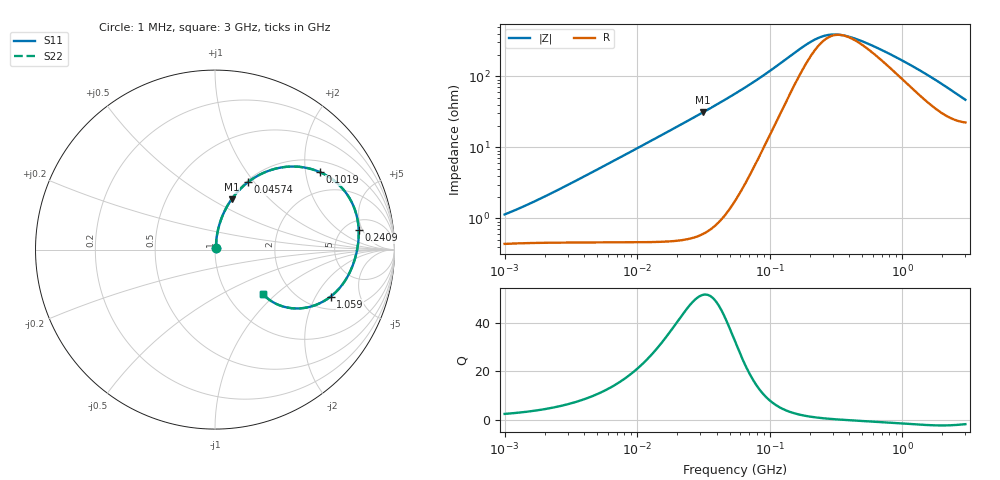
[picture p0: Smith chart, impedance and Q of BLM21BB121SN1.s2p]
! BLM21BB121SN1
# Hz S RI R 50
!Freq.(Hz) S11(Real) S11(Imag) S21(Real) S21(Imag) S12(Real) S12(Imag) S22(Real) S22(Imag)
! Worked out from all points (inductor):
!   401 points, 1 MHz to 3 GHz, reference 50 ohm
!   read as one part in series: L = 159 nH near 1.323 MHz
!   highest Q = 51.5 at 31.27 MHz (marker M1), where L = 158 nH
!   self-resonance near 349.5 MHz
!   S11 on the Smith chart (normalised r, x): 1 MHz: 1.01, +0.02; 45.74 MHz: 1.02, +0.93; 101.9 MHz: 1.32, +2.41; 240.9 MHz: 6.75, +4.21; 1.059 GHz: 2.65, -2.69; 3 GHz: 1.45, -0.82
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1000000  0.00447 0.0104  0.9955 -0.0104  0.9955 -0.0104  0.00447 0.0104
1716745  0.00479 0.0169  0.9952 -0.0169  0.9952 -0.0169  0.00479 0.0169
3823119  0.00593 0.0368  0.9941 -0.0368  0.9941 -0.0368  0.00593 0.0368
8017732  0.0105 0.0766  0.9895 -0.0766  0.9895 -0.0766  0.0105 0.0766
1.461624e7  0.0242 0.138  0.9758 -0.138  0.9758 -0.138  0.0242 0.138
3.127247e7  0.0921 0.2796  0.9079 -0.2796  0.9079 -0.2796  0.0921 0.2796
4.574308e7  0.1838 0.3757  0.8162 -0.3757  0.8162 -0.3757  0.1838 0.3757
5.477226e7  0.2512 0.4185  0.7488 -0.4185  0.7488 -0.4185  0.2512 0.4185
7.697298e7  0.4241 0.4628  0.5759 -0.4628  0.5759 -0.4628  0.4241 0.4628
1.018679e8  0.5852 0.4314  0.4148 -0.4314  0.4148 -0.4314  0.5852 0.4314
1.460522e8  0.7381 0.3042  0.2619 -0.3042  0.2619 -0.3042  0.7381 0.3042
2.094008e8  0.7958 0.1576  0.2042 -0.1576  0.2042 -0.1576  0.7958 0.1576
2.408952e8  0.8007 0.1084  0.1993 -0.1084  0.1993 -0.1084  0.8007 0.1084
3.002264e8  0.7982 0.041  0.2018 -0.041  0.2018 -0.041  0.7982 0.041
3.741707e8  0.7884 -0.0174  0.2116 0.0174  0.2116 0.0174  0.7884 -0.0174
5.051982e8  0.7667 -0.0899  0.2333 0.0899  0.2333 0.0899  0.7667 -0.0899
8.005644e8  0.7072 -0.1982  0.2928 0.1982  0.2928 0.1982  0.7072 -0.1982
1.059487e9  0.6447 -0.2613  0.3553 0.2613  0.3553 0.2613  0.6447 -0.2613
1.430499e9  0.5476 -0.3133  0.4524 0.3133  0.4524 0.3133  0.5476 -0.3133
1.818868e9  0.4506 -0.3279  0.5494 0.3279  0.5494 0.3279  0.4506 -0.3279
2.266846e9  0.359 -0.31  0.641 0.31  0.641 0.31  0.359 -0.31
3e9  0.2657 -0.2464  0.7343 0.2464  0.7343 0.2464  0.2657 -0.2464
